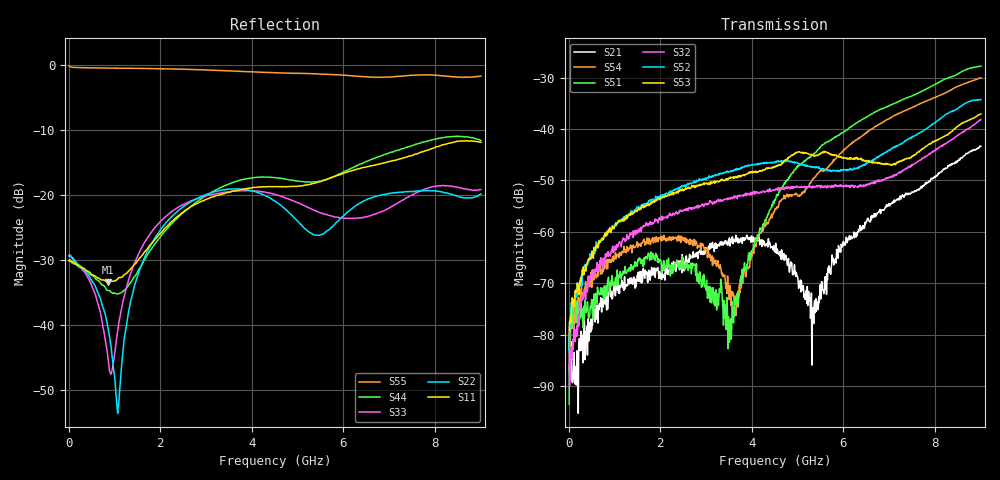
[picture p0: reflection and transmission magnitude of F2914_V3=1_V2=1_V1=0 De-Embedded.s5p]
! Integrated Device Technology
! Corporate Headquarters
! 6024 Silver Creek Valley Road
! San Jose, CA 95138  USA
! Phone:  1-408-284-8200
! Toll Free:  1-800-223-1366
! Webpage:  http://www.idt.com/
! Timing and RF Division
! 515 Groton Road, Suite 102
! Westford, MA 01886-6024
! Device:  F2914
! Description: High Reliability SP4T RF Switch
! Frequency:  0.05 -  8.GHz
! Package:  4x4 mm Thin QFN Plastic Package: 24 pin
! Ports:  5 RF,  5 DC
!  Pin  1  = GND
!  Pin  2  = GND
!  Pin  3  = GND
!  Pin  4  = GND
!  Pin  5  = RF4  =  Port 4
!  Pin  6  = GND
!  Pin  7  = GND
!  Pin  8  = RF3  =  Port 3
!  Pin  9  = GND
!  Pin 10  = GND
!  Pin 11  = RF2  =  Port 2
!  Pin 12  = GND
!  Pin 13  = GND
!  Pin 14  = RF1  =  Port 1
!  Pin 15  = GND
!  Pin 16  = Vcc
!  Pin 17  = V1
!  Pin 18  = V2
!  Pin 19  = V3
!  Pin 20  = VSSext
!  Pin 21  = GND
!  Pin 22  = RFC  =  Port 5
!  Pin 23  = GND
!  Pin 24  = GND
! Voltage:  VDD  =  +3.30 Volts
!  VSSEXT =  0.00 Volts
! Current:  IDD  = 330  uA
! State:  All OFF
! V1:  Logic LOW
! V2:  Logic HIGH
! V3:  Logic HIGH
! Data:  The device was measured on the F291x evaluation board which has
!  individual transmission lines to the RF pins.  Data was collected
!  using a calibrated network analyzer.  The input lines were
!  modeled using Automatic Fixture Removal (AFR) from Keysight.
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# Hz S  dB  R 50
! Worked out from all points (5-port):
!   900 points, 10 MHz to 9 GHz, reference 50 ohm
!   strongest paths, dB at 10 MHz, 2.26 GHz, 4.51 GHz, 6.76 GHz, 9 GHz:
!     S53: -79.3, -52.6, -47.2, -46.6, -37.0
!     S52: -83.0, -52.2, -46.3, -45.4, -34.3
!     S32: -85.2, -56.9, -51.8, -50.1, -38.2
!     S51: -93.5, -66.6, -53.8, -36.4, -27.8
!     S54: -79.7, -61.2, -55.4, -39.1, -30.0
!     S21: -79.7, -66.4, -64.0, -56.2, -43.4
!   lowest |S11| = -33.3 dB at 850 MHz (marker M1), VSWR 1.04, Z = 48.6 + j1.59 ohm
!   |S11| at or under -10 dB: start of sweep to end of sweep
